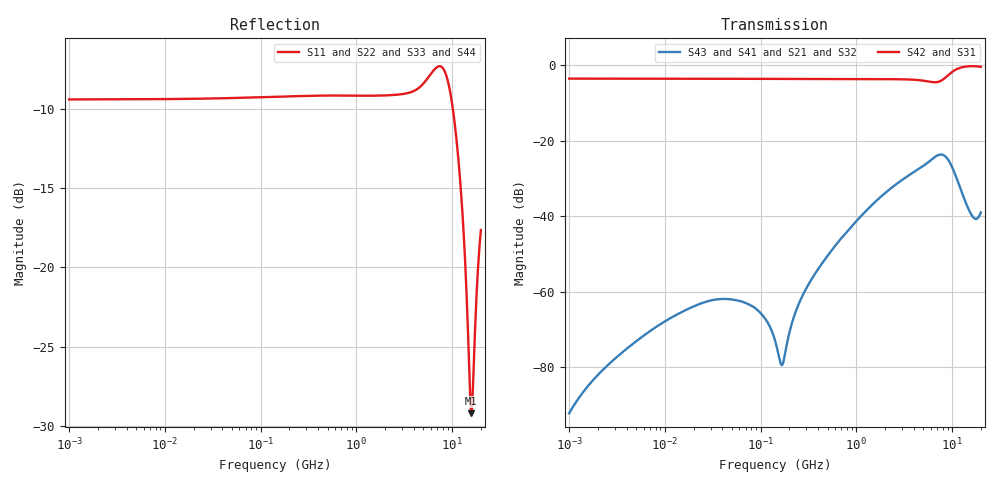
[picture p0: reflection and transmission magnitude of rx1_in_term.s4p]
! Created Mon Mar 13 11:20:10 2017
# hz S ma R 50
! 4 Port Network Data from SP1.SP block
! freq  magS11  angS11  magS12  angS12  magS13  angS13  magS14  angS14
!  magS21  angS21  magS22  angS22  magS23  angS23  magS24  angS24
!  magS31  angS31  magS32  angS32  magS33  angS33  magS34  angS34
!  magS41  angS41  magS42  angS42  magS43  angS43  magS44  angS44
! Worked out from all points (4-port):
!   861 points, 1 MHz to 20 GHz, reference 50 ohm
!   strongest paths, dB at 1 MHz, 11.89 MHz, 141.4 MHz, 1.682 GHz, 20 GHz:
!     S42: -3.6, -3.6, -3.7, -3.7, -0.5
!     S31: -3.6, -3.6, -3.7, -3.7, -0.5
!     S43: -92.1, -66.7, -72.8, -35.5, -39.0
!     S41: -92.1, -66.7, -72.8, -35.5, -39.0
!     S21: -92.1, -66.7, -72.8, -35.5, -39.0
!     S32: -92.2, -66.7, -73.3, -35.5, -39.0
!   lowest |S11| = -29.2 dB at 15.89 GHz (marker M1), VSWR 1.07, Z = 46.6 + j0.0247 ohm
!   |S11| at or under -10 dB: 10.19 GHz to end of sweep
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1000000  0.3382 -178.7  2.469e-05 158.2  0.6619 -0.6  2.469e-05 158.2
         2.474e-05 158.2  0.3382 -178.7  2.474e-05 158.2  0.6619 -0.6
         0.6619 -0.6  2.469e-05 158.2  0.3382 -178.7  2.469e-05 158.2
         2.474e-05 158.2  0.6619 -0.6  2.474e-05 158.2  0.3382 -178.7
4.030737e7  0.3411 -179.5  0.0007931 18.5  0.6589 -0.2  0.0007931 18.5
            0.0008056 18.8  0.3406 -179.5  0.0008056 18.8  0.6594 -0.3
            0.6589 -0.2  0.0007931 18.5  0.3411 -179.5  0.0007931 18.5
            0.0008056 18.8  0.6594 -0.3  0.0008056 18.8  0.3406 -179.5
1.66162e8  0.345 -179.4  0.0001142 60.9  0.655 -0.3  0.0001142 60.9
           0.0001069 51.7  0.3451 -179.4  0.0001069 51.7  0.6549 -0.3
           0.655 -0.3  0.0001142 60.9  0.345 -179.4  0.0001142 60.9
           0.0001069 51.7  0.6549 -0.3  0.0001069 51.7  0.3451 -179.4
2.34859e9  0.3491 178.5  0.02403 49.3  0.6511 0.8  0.02403 49.3
           0.02397 49.5  0.3495 178.6  0.02397 49.5  0.6506 0.8
           0.6511 0.8  0.02403 49.3  0.3491 178.5  0.02403 49.3
           0.02397 49.5  0.6506 0.8  0.02397 49.5  0.3495 178.6
9.035399e9  0.3867 142.9  0.05662 -138.1  0.7301 18.6  0.05662 -138.1
            0.05666 -138.0  0.3886 143.0  0.05666 -138.0  0.7282 18.7
            0.7301 18.6  0.05662 -138.1  0.3867 142.9  0.05662 -138.1
            0.05666 -138.0  0.7282 18.7  0.05666 -138.0  0.3886 143.0
1.588569e10  0.03471 179.6  0.01055 91.3  0.9653 0.0  0.01055 91.3
             0.01055 91.4  0.03344 175.8  0.01055 91.4  0.9667 0.1
             0.9653 0.0  0.01055 91.3  0.03471 179.6  0.01055 91.3
             0.01055 91.4  0.9667 0.1  0.01055 91.4  0.03344 175.8
2e10  0.1311 -118.8  0.01127 -6.6  0.9439 -7.0  0.01127 -6.6
      0.01125 -6.6  0.1297 -117.1  0.01125 -6.6  0.9479 -7.0
      0.9439 -7.0  0.01127 -6.6  0.1311 -118.8  0.01127 -6.6
      0.01125 -6.6  0.9479 -7.0  0.01125 -6.6  0.1297 -117.1
